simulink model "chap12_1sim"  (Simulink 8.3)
settings: Solver=ode45  StartTime=0.0  StopTime=10  RelTol=1e-3

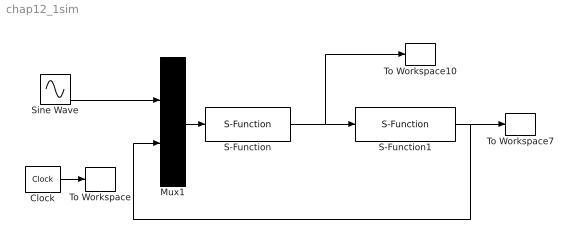
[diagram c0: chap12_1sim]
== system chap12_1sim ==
  Clock : Clock
  Mux1 : Mux  Inputs=2
  S-Function : S-Function  FunctionName=chap12_1ctrl  EnableBusSupport=off
  S-Function1 : S-Function  FunctionName=chap12_1plant  EnableBusSupport=off
  Sine Wave : Sin  SampleTime=0
  To Workspace : ToWorkspace  VariableName=t  SampleTime=-1
  To Workspace10 : ToWorkspace  VariableName=ut  SampleTime=-1
  To Workspace7 : ToWorkspace  VariableName=y  SampleTime=-1
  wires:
  Mux1/1 -> S-Function/1
  S-Function/1 -> S-Function1/1, To Workspace10/1
  S-Function1/1 -> Mux1/2, To Workspace7/1
  Sine Wave/1 -> Mux1/1
  Clock/1 -> To Workspace/1
